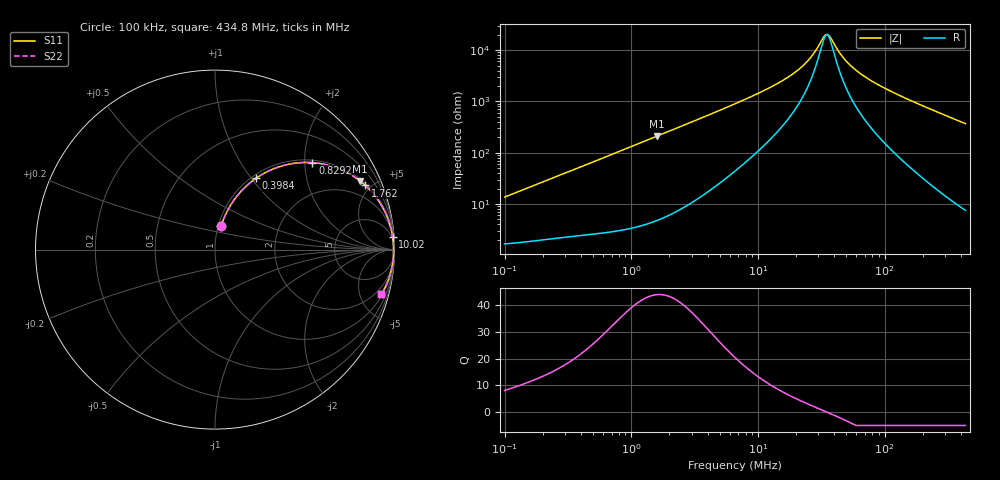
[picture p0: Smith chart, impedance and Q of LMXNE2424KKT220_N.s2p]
! LMXNE2424KKT220_N  S-PARAMETER MODEL  ( General Type )
! Model Generated by TAIYO YUDEN Corporation (http://www.ty-top.com)
! Version 1.0
! TAIYO YUDEN Control No. 191023NI43SB-FBB
! Copyright(c) 2019 TAIYO YUDEN CO.,LTD. All Rights Reserved.
! Product Description (link to TY-COMPAS)
! https://ds.yuden.co.jp/TYCOMPAS/or/detail?pn=LMXNE2424KKT220MN&u=M
! Products Name : Inductors
! Characteristics :
!  Inductance : 22 uH , SRF(min) : 22 MHz , DC Resistance(max) : 1.764 Ohm
!  Rated Current : Saturation :390 mA , Temp Rise : 300 mA
!  Case Size : 2.4 x 2.4 / 0.094 x 0.094 [mm/inch] , Thickness : 1 / 0.039 [mm/inch]
!  (Conditions: Temperature = 25 degC , DC Bias Current/Voltage = 0A / 0V)
! External Node Assignments :
!  1  o---GGG---o  2
! GND o---------o GND
! Frequency Range : 0.1MHz  -  434.768421MHz  [ 402 STEP ]
# MHz S RI R 50
! Freq[MHz].  S11 Real  S11 Imag  S21 Real  S21 Imag  S12 Real  S12 Imag  S22 Real  S22 Imag
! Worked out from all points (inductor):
!   401 points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, 100 kHz to 434.8 MHz, reference 50 ohm
!   read as one part in series: L = 21.5 uH near 104.3 kHz
!   highest Q = 44 at 1.587 MHz (marker M1), where L = 21 uH
!   self-resonance near 34.49 MHz
!   S11 on the Smith chart (normalised r, x): 100 kHz: 1.03, +0.27; 398.4 kHz: 1.05, +1.06; 829.2 kHz: 1.06, +2.19; 1.762 MHz: 1.11, +4.64; 10.02 MHz: 3, +29; 434.8 MHz: 1.15, -7.37
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0.1  0.0336 0.1288  0.9664 -0.1288  0.9664 -0.1288  0.0336 0.1288
0.221633  0.0964 0.2625  0.9036 -0.2625  0.9036 -0.2625  0.0964 0.2625
0.398394  0.2286 0.3976  0.7714 -0.3976  0.7714 -0.3976  0.2286 0.3976
0.406826  0.2355 0.4022  0.7645 -0.4022  0.7645 -0.4022  0.2355 0.4022
0.829202  0.5432 0.4843  0.4568 -0.4843  0.4568 -0.4843  0.5432 0.4843
1.587176  0.8085 0.3823  0.1915 -0.3823  0.1915 -0.3823  0.8085 0.3823
1.65507  0.8208 0.3723  0.1792 -0.3723  0.1792 -0.3723  0.8208 0.3723
1.762395  0.8381 0.3572  0.1619 -0.3572  0.1619 -0.3572  0.8381 0.3572
3.102314  0.9386 0.2268  0.0614 -0.2268  0.0614 -0.2268  0.9386 0.2268
6.733248  0.9831 0.1064  0.0169 -0.1064  0.0169 -0.1064  0.9831 0.1064
10.02402  0.99 0.0687  0.00998 -0.0687  0.00998 -0.0687  0.99 0.0687
18.39991  0.994 0.0297  0.00596 -0.0297  0.00596 -0.0297  0.994 0.0297
22.68674  0.9946 0.0193  0.00541 -0.0193  0.00541 -0.0193  0.9946 0.0193
26.82484  0.9949 0.0116  0.00514 -0.0116  0.00514 -0.0116  0.9949 0.0116
33.07453  0.995 0.00249  0.00496 -0.00249  0.00496 -0.00249  0.995 0.00249
35.96468  0.9951 -0.00112  0.00493 0.00112  0.00493 0.00112  0.9951 -0.00112
46.24065  0.995 -0.0121  0.005 0.0121  0.005 0.0121  0.995 -0.0121
55.83221  0.9948 -0.0209  0.00523 0.0209  0.00523 0.0209  0.9948 -0.0209
73.30408  0.9941 -0.035  0.00595 0.035  0.00595 0.035  0.9941 -0.035
109.1303  0.9917 -0.0605  0.00833 0.0605  0.00833 0.0605  0.9917 -0.0605
222.432  0.9773 -0.1324  0.0227 0.1324  0.0227 0.1324  0.9773 -0.1324
434.7684  0.927 -0.2501  0.073 0.2501  0.073 0.2501  0.927 -0.2501
